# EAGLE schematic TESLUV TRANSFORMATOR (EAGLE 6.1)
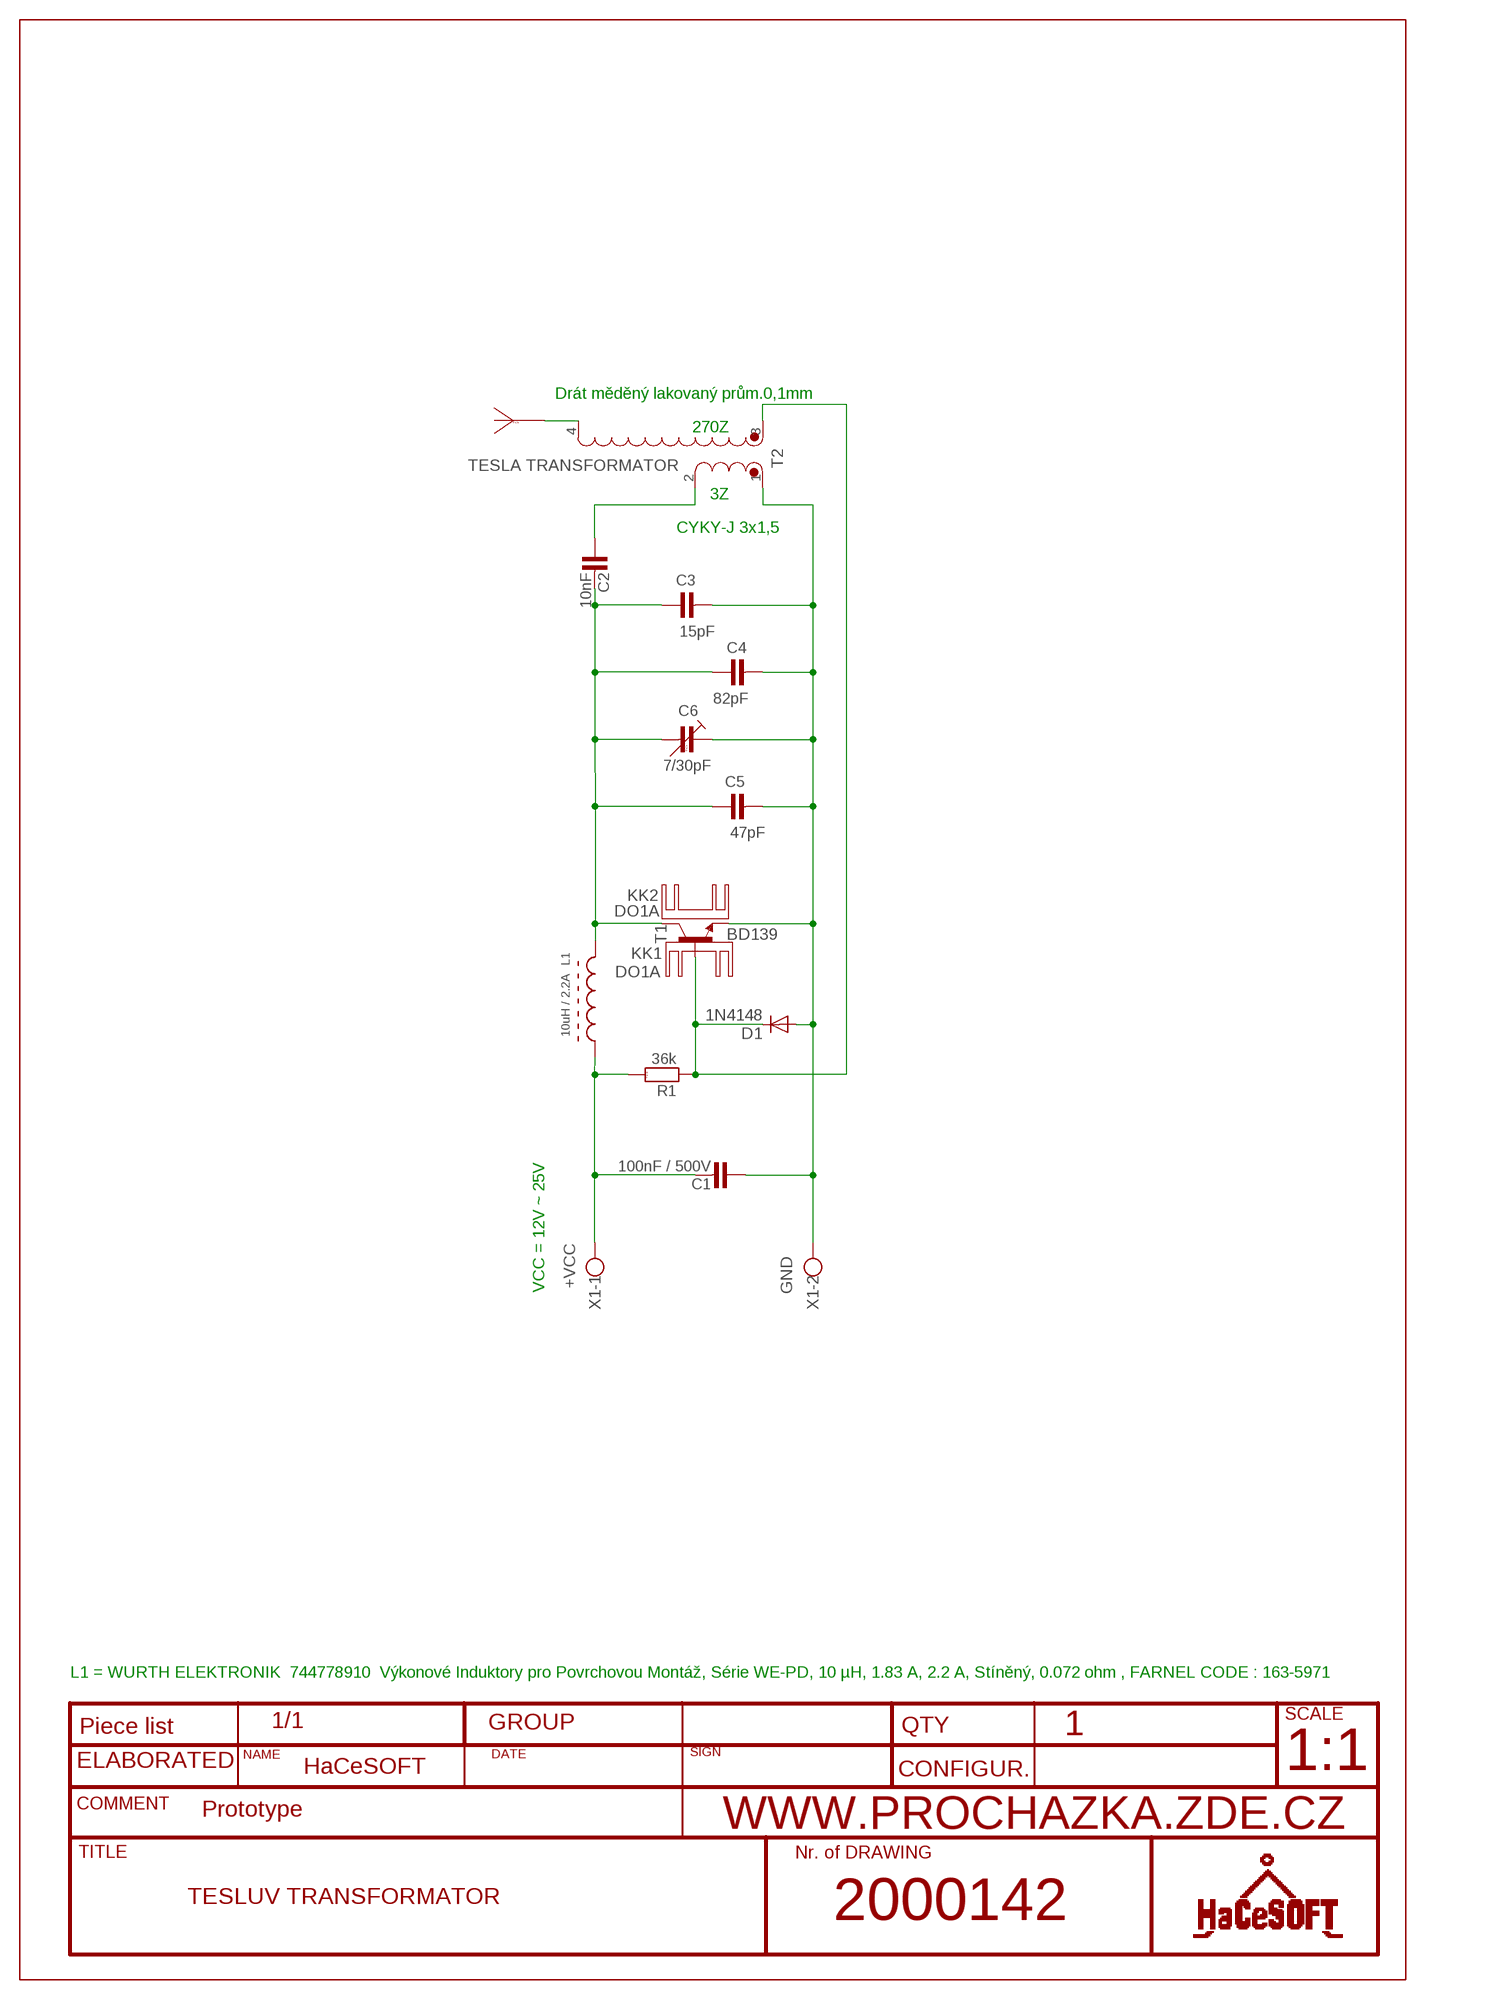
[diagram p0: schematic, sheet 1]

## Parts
ANT1  ANTENA  [PAD_1]
C1  100nF / 500V  C-KERAMIK_5  [C-5]
C2  10nF  C-KERAMIK_5  [C-5]
C3  15pF  C-KERAMIK_5  [C-5]
C4  82pF  C-KERAMIK_5  [C-5]
C5  47pF  C-KERAMIK_5  [C-5]
C6  7/30pF  CKT  [CKT]
D1  1N4148  [DO35-10]
KK1  DO1A  DO2A-L  [D02A-L]
KK2  DO1A  DO2A-L  [D02A-L]
L1  10uH / 2.2A  INDUCTOR  [INDUCTOR10UH]
R1  36k  R_5  [R-5]
T1  BD139  [TO126]
T2  TESLA TRANSFORMATOR  TRANSFORMATOR  [TRANSFORMATOR]
X1  W237-102  [W237-102]

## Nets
+VCC: C1.2 L1.P$1 R1.2 X1.1
GND: C1.1 C3.2 C4.2 C5.2 C6.1 D1.A T1.1(E) T2.1 X1.2
N$1: C4.1
N$2: C6.3
N$3: C5.1
N$4: T1.2(C)
N$5: C2.1 T2.2
N$6: D1.C R1.1 T1.3(B) T2.3
N$7: C2.2 C3.1 L1.P$2
N$10: ANT1.1 T2.4
Unconnected: C6.2

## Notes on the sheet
- Drát měděný lakovaný prům.0,1mm
- 270Z
- 3Z
- CYKY-J 3x1,5
- VCC = 12V ~ 25V
- L1 = WURTH ELEKTRONIK  744778910  Výkonové Induktory pro Povrchovou Montáž, Série WE-PD, 10 µH, 1.83 A, 2.2 A, Stíněný, 0.072 ohm , FARNEL CODE : 163-5971
- 1
- HaCeSOFT | 1:1
- Prototype
- 2000142

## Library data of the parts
ANT1 = #PaJa_15:ANTENA: SCH symbol - Anteny + pajeci bod na DPS
C1-C5 = #hacesoft:C-KERAMIK: Kondenzator - keramicky
C6 = #PaJa_30:CKT: Kapacitni trimr
D1 = #hacesoft:1N4148: DIODE
KK1 KK2 = heatsink:DO2A-L
L1 = #hacesoft:INDUCTOR
R1 = #PaJa_30:R: Rezistor
T1 = transistor:BD139: NPN TRANSISTOR
T2 = e-spulen-transformatoren:TRANSFORMATOR: Transformator
X1 = con-wago-500:W237-102: WAGO SCREW CLAMP; MPN: 237-102; OC_FARNELL: unknown; OC_NEWARK: 70K9898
